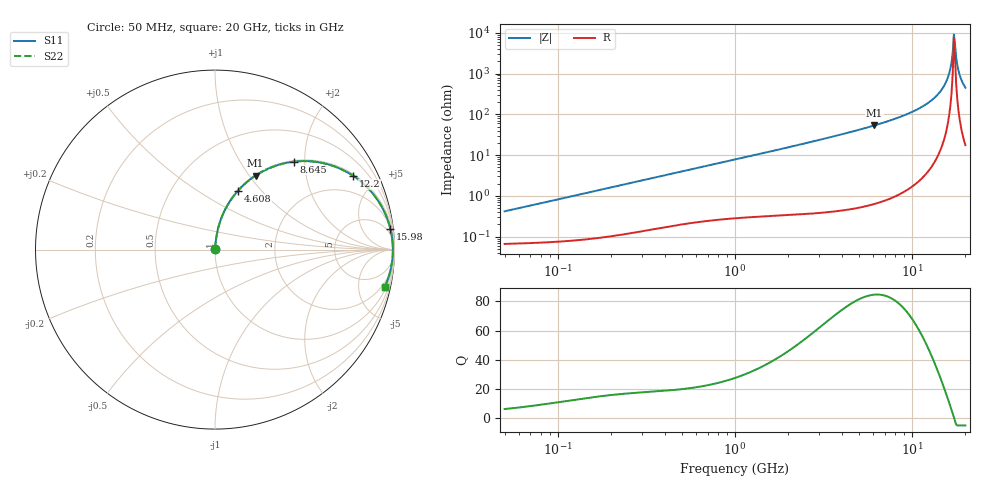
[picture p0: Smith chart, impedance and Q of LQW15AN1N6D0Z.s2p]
!Murata Part Number: LQW15AN1N6D0Z
!These Parameters are Measured in Series Mode Connection
!  o--[Z]--o
!Port1  Port2
!  o-------o
!Freq. Start=50[MHz] Stop=20[GHz], 401[Steps]
# Hz S RI R 50
!Freq.(Hz) S11(Real) S11(Imag) S21(Real) S21(Imag) S12(Real) S12(Imag) S22(Real) S22(Imag)
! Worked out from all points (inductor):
!   401 points, 50 MHz to 20 GHz, reference 50 ohm
!   read as one part in series: L = 1.31 nH near 51.52 MHz
!   highest Q = 84.6 at 6.125 GHz (marker M1), where L = 1.39 nH
!   self-resonance near 17.22 GHz
!   S11 on the Smith chart (normalised r, x): 50 MHz: 1.00, +0.01; 4.608 GHz: 1.01, +0.76; 8.645 GHz: 1.02, +1.76; 12.2 GHz: 1.08, +3.72; 15.98 GHz: 2, +17; 20 GHz: 1.35, -9.03
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5e7  0.000681 0.00414  0.9993 -0.00414  0.9993 -0.00414  0.000681 0.00414
1.364002e8  0.000961 0.0111  0.999 -0.0111  0.999 -0.0111  0.000961 0.0111
3.721004e8  0.00249 0.0296  0.9975 -0.0296  0.9975 -0.0296  0.00249 0.0296
1e9  0.00879 0.0769  0.9912 -0.0769  0.9912 -0.0769  0.00879 0.0769
2.728004e9  0.0472 0.2036  0.9528 -0.2036  0.9528 -0.2036  0.0472 0.2036
4.608136e9  0.1292 0.3292  0.8708 -0.3292  0.8708 -0.3292  0.1292 0.3292
6.125241e9  0.226 0.4124  0.774 -0.4124  0.774 -0.4124  0.226 0.4124
7.442007e9  0.3302 0.4643  0.6698 -0.4643  0.6698 -0.4643  0.3302 0.4643
8.644534e9  0.4384 0.4898  0.5616 -0.4898  0.5616 -0.4898  0.4384 0.4898
1.220001e10  0.7711 0.4101  0.2289 -0.4101  0.2289 -0.4101  0.7711 0.4101
1.438523e10  0.9198 0.2545  0.0802 -0.2545  0.0802 -0.2545  0.9198 0.2545
1.527346e10  0.9574 0.178  0.0426 -0.178  0.0426 -0.178  0.9574 0.178
1.597544e10  0.977 0.1156  0.023 -0.1156  0.023 -0.1156  0.977 0.1156
1.646126e10  0.9855 0.0723  0.0145 -0.0723  0.0145 -0.0723  0.9855 0.0723
1.696185e10  0.9901 0.0282  0.00986 -0.0282  0.00986 -0.0282  0.9901 0.0282
1.721783e10  0.991 0.006  0.00904 -0.006  0.00904 -0.006  0.991 0.006
1.747767e10  0.9908 -0.0162  0.00921 0.0162  0.00921 0.0162  0.9908 -0.0162
1.774144e10  0.9896 -0.0384  0.0104 0.0384  0.0104 0.0384  0.9896 -0.0384
1.828096e10  0.9843 -0.0825  0.0157 0.0825  0.0157 0.0825  0.9843 -0.0825
1.855685e10  0.9802 -0.1042  0.0198 0.1042  0.0198 0.1042  0.9802 -0.1042
1.940974e10  0.9623 -0.1674  0.0377 0.1674  0.0377 0.1674  0.9623 -0.1674
2e10  0.946 -0.2074  0.054 0.2074  0.054 0.2074  0.946 -0.2074
